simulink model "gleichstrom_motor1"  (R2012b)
settings: Solver=ode45  StartTime=0.0  StopTime=10.0  RelTol=1e-3
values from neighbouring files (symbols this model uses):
  cj = 10    [gleichstrom_motor_1.m]    (also in unwucht_rueckw_1.m = 0.1)
  J = 10    [gleichstrom_motor_1.m]    (also in unwucht_rueckw_1.m)
  km = 10    [gleichstrom_motor_1.m]    (also in unwucht_rueckw_1.m)
  L = 1    [gleichstrom_motor_1.m]    (also in suspension_1.m = 3; suspension_2.m = 3; suspension_3.m = 3; suspension_4.m = 3)
  R = 0.1    [gleichstrom_motor_1.m]    (also in unwucht_rueckw_1.m; vibration_control_1.m = 15; vibration_control_2.m = 15; vibration_control_3.m = 15)
  U = fft(u)    [feder_masse_13.m]    (also in feder_masse_14.m; gleichstrom_motor_1.m = 100; unwucht_rueckw_1.m = 50)

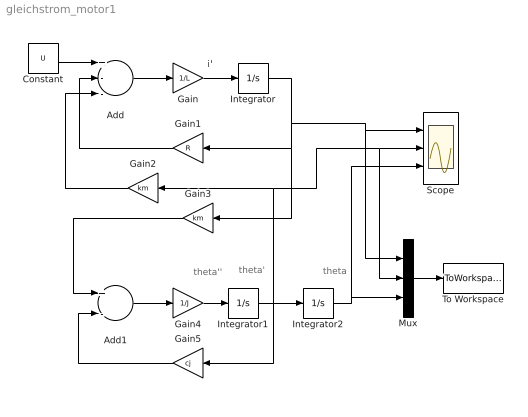
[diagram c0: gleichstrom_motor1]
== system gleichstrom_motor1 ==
  note: theta''
  note: theta'
  note: theta
  note: i
  note: i'
  Add : Sum  Inputs=+--
  Add1 : Sum  Inputs=+-
  Constant : Constant  Value=U
  Gain : Gain  Gain=1/L
  Gain1 : Gain  Gain=R
  Gain2 : Gain  Gain=km
  Gain3 : Gain  Gain=km
  Gain4 : Gain  Gain=1/J
  Gain5 : Gain  Gain=cj
  Integrator : Integrator
  Integrator1 : Integrator
  Integrator2 : Integrator
  Mux : Mux  Inputs=3
  Scope : Scope  NumInputPorts=3
  To Workspace : ToWorkspace  VariableName=xy  SampleTime=-1  SaveFormat=Structure With Time
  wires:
  Constant/1 -> Add/1
  Add/1 -> Gain/1
  Gain/1 -> Integrator/1
  Gain1/1 -> Add/2
  Integrator/1 -> Mux/1, Scope/1, Gain3/1, Gain1/1
  Gain2/1 -> Add/3
  Gain3/1 -> Add1/1
  Add1/1 -> Gain4/1
  Gain4/1 -> Integrator1/1
  Integrator2/1 -> Mux/3, Scope/3
  Gain5/1 -> Add1/2
  Integrator1/1 -> Gain5/1, Mux/2, Scope/2, Gain2/1, Integrator2/1
  Mux/1 -> To Workspace/1
